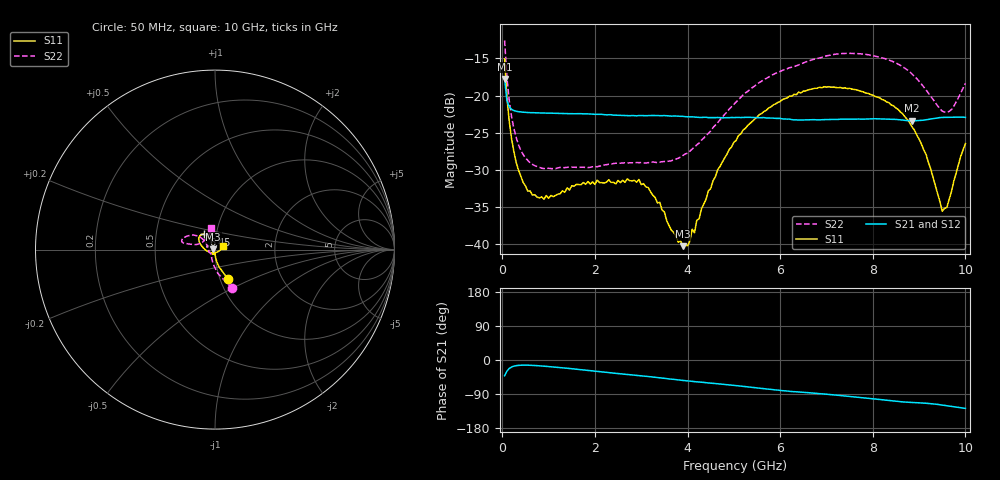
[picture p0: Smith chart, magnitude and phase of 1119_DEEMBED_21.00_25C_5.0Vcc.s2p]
!Hittite Microwave Corp.
!Digital Attenuator/PhaseShifter Rev 1.4.0
!Filename: C:\DATA\DATA\1119_DEEMBED_21.00_25C_5.0Vcc.s2p
!VNA ID: Agilent Technologies,N5224A,MY51441122,A.10.45.03
!Device type:
!2 Port Calibration.
!Temp(C): 25
!Lot Number:
!Serial Number:
!Operator:
!Misc:
!Attenuator:  21.000
# GHZ S DB R 50.0
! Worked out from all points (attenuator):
!   200 points, 50 MHz to 10 GHz, reference 50 ohm
!   highest |S21| = -17.77 dB at 50 MHz (marker M1); lowest = -23.4 dB at 8.85 GHz (marker M2)
!   lowest |S11| = -40.3 dB at 3.9 GHz (marker M3), VSWR 1.02, Z = 49 + j0.0684 ohm
!   |S11| at or under -10 dB: start of sweep to end of sweep
!   |S22| runs from -29.8 to -12.6 dB; largest |S21 - S12| = 0.00026
!   S11 on the Smith chart (normalised r, x): 50 MHz: 1.09, -0.36; 6.45 GHz: 0.87, +0.15; 10 GHz: 1.09, +0.04
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0.05  -15.06 -66.5  -17.77 -41.7  -17.77 -41.7  -12.59 -66.4
0.1  -20.28 -77.4  -20.70 -29.5  -20.70 -29.5  -17.55 -83.4
0.2  -25.81 -84.4  -21.86 -18.5  -21.86 -18.5  -22.83 -100.1
0.35  -30.04 -88.0  -22.17 -14.2  -22.17 -14.2  -26.63 -114.0
0.55  -32.85 -92.6  -22.28 -13.7  -22.28 -13.7  -28.72 -125.6
0.9  -33.94 -98.6  -22.35 -16.3  -22.35 -16.3  -29.82 -134.8
1.75  -31.70 -113.0  -22.46 -26.2  -22.46 -26.2  -29.64 -139.5
2.95  -31.29 -114.1  -22.69 -41.0  -22.70 -41.0  -29.03 -158.5
3.4  -34.36 -127.9  -22.70 -47.0  -22.71 -47.0  -28.97 -171.9
3.9  -40.26 175.9  -22.80 -53.9  -22.81 -53.9  -28.07 168.4
4.15  -38.47 136.4  -22.89 -57.1  -22.89 -57.1  -26.94 157.6
4.65  -29.98 113.2  -22.95 -62.8  -22.97 -62.8  -23.65 143.1
5.05  -26.04 113.0  -22.95 -67.5  -22.97 -67.5  -20.84 139.6
5.55  -22.56 117.0  -22.99 -74.2  -23.00 -74.2  -18.25 141.9
6.45  -19.65 125.8  -23.29 -84.7  -23.30 -84.7  -15.73 151.4
6.7  -19.10 130.4  -23.25 -87.2  -23.26 -87.2  -15.17 154.5
8.35  -20.97 158.3  -23.18 -106.8  -23.18 -106.8  -15.22 168.0
8.85  -24.23 174.4  -23.40 -112.1  -23.41 -112.1  -17.12 167.6
9.15  -27.89 -162.9  -23.26 -114.1  -23.28 -114.1  -19.24 165.0
9.5  -35.56 -93.0  -22.94 -118.9  -22.96 -118.9  -22.09 144.0
9.6  -35.06 -54.6  -22.93 -120.7  -22.94 -120.7  -22.24 132.9
10  -26.46 21.9  -22.94 -127.7  -22.94 -127.7  -18.35 99.5
